(* Logix 5000 Rung export; software revision 16.03 *)

MODULES
   Local : vendor None type None code None
   mcm : vendor None type None code None
END_MODULES

TYPE MCMCONTROL :   // Stores control registers used by the processor to request special tasks from the module.
STRUCT
   WarmBoot : BOOL;   // Warm Boot
   ColdBoot : BOOL;   // Cold Boot
   SlaveControl : MCMSlaveControl;
   CmdControl : MCMCmdControl;   // Allows for a disabled command to be sent to a device (MASTER)
   EventCmd : MCMEventCmd;   // Allows a command defined in ladder to be sent to a device (MASTER)
   SlavePollStat : MCMSlavePollStatus;   // Request slave poll status for the port (MASTER).
   Passthru : MCMPassthru;   // Contains PassThru objects required when PortX.Type is set to a value between 2-4.
END_STRUCT
END_TYPE

TYPE MCMDATA :   // Contains Read Data (data read from the module to the processor) and Write Data (data written from the processor to the module)
STRUCT
   ReadData : INT[600];   // Data read from the module to the processor
   WriteData : INT[600];   // Data written from the processor to the module
END_STRUCT
END_TYPE

TYPE MCMModule :   // This object contains the information used to define the data movement between the module and the processor.
STRUCT
   WriteStartReg : INT;   // Start reg to transfer from PLC to module
   WriteRegCnt : INT;   // Number of registers to write from PLC
   ReadStartReg : INT;   // Start reg to transfer from module to PLC
   ReadRegCnt : INT;   // Number of registers to transfer from module
   BPFail : INT;   // Determines module operation if BP fails 0=continue,>0=number of retries before comm shutdown
   ErrStatPtr : INT;   // Internal DB start register for status data (-1=Ignore)
END_STRUCT
END_TYPE

TYPE MCMCONFIG :   // This object contains the data types that apply to the configuration of the module.
STRUCT
   ModDef : MCMModule;   // Module Defintion
   Port1 : MCMPort;   // Port 1 configuration settings
   Port2 : MCMPort;   // Port 2 configuration settings
   Port1MasterCmd : MCMCmd[325];   // Master commands for Port 1 (ignore if port is configured for slave mode)
   Port2MasterCmd : MCMCmd[325];   // Master commands for Port 2 (ignore if port is configured for slave mode)
END_STRUCT
END_TYPE

TYPE MCMCmdControl :   // Command Control
STRUCT
   TriggerCmdCntrl : BOOL;   // Trigger command control. User application will activate this trigger
   NumberOfCommands : INT;   // Number of commands per block (1 to 6)
   PortNumber : INT;   // MVI56-MCM Port Number of master port (1 or 2)
   CommandIndex : INT[6];   // Stores the command indexes for command control
   CmdsAddedToQueue : INT;   // Number of commands added to queue
   CmdControlBlockID : INT;   // Temporary variable to calculate control block ID
   CmdCntrlPending : BOOL;   // Auxiliary control command - prevents a second request before acknowledgment is received
END_STRUCT
END_TYPE

TYPE MCMSlaveControl :   // Special block processing for Slave Control.
STRUCT
   TriggerSlaveControl : BOOL;   // Trigger to Enable or Disable Slaves
   PortNumber : INT;   // Slave Address
   NumberOfSlaves : INT;   // Number of Slaves
   BlockNumber : INT;   // Block ID number
   SlaveIndexes : INT[200];   // Slave Indexes
   NumberOfSlavesProcessed : INT;   // Number of Slaves processed
   EnableSlaves : BOOL;   // Set 0 to Disable or 1 to Enable Slaves
END_STRUCT
END_TYPE

TYPE MCMModuleDef :   // This object contains the data types that apply to the operation of the module.
STRUCT
   CONFIG : MCMCONFIG;   // Module and port configuration
   DATA : MCMDATA;   // Modbus data transferred between module and processor
   STATUS : MCMSTATUS;   // Status information in each read block
   CONTROL : MCMCONTROL;   // Optional requests from the processor to the module
   UTIL : MCMUTIL;   // Variables for internal ladder usage - should not be accessed by user application
END_STRUCT
END_TYPE

TYPE MCMPort :   // The serial port configuration for the MVI56MCM module.
STRUCT
   Enabled : INT;   // O=Port Disabled,1=Port Enabled
   Type : INT;   // 0=Master, 1=Slave, 2=Slave: pass-through, 3=Slave: formatted pass-through/data swapped, 4=Slave: form. pass-through
   FloatFlag : INT;   // 0=No floating-point data, 1=Use floating-point data
   FloatStart : INT;   // Register offset in message for floating-point data
   FloatOffset : INT;   // Internal DB offset to start of floating-point data
   Protocol : INT;   // 0=Modbus RTU, 1=Modbus ASCII
   Baudrate : INT;   // Baudrate for port (110 to 115.2K)
   Parity : INT;   // 0=None, 1=Odd, 2=Even, 3=Mark, 4=Space
   DataBits : INT;   // 5 to 8 data bits
   StopBits : INT;   // 1 or 2 stop bits
   RTSOn : INT;   // 0-65535 mSec delay before data
   RTSOff : INT;   // 0-65535 mSec delay after data
   MinResp : INT;   // 0-65535 mSec minimum time before response to request
   UseCTS : INT;   // 0=No, 1=Yes to use CTS modem line
   SlaveID : INT;   // 1-255 Modbus Node Address (Slave)
   BitInOffset : INT;   // Internal DB offset to bit input data (Slave)
   WordInOffset : INT;   // Internal DB offset to word input data (Slave)
   OutOffset : INT;   // Internal DB offset to bit output data (Slave)
   HoldOffset : INT;   // Internal DB offset to holding register data (Slave)
   CmdCount : INT;   // Command list count (Master)
   MinCmdDelay : INT;   // 0-65535 mSec minimum time between each command (Master)
   CmdErrPtr : INT;   // Internal DB location to place command error list (Master)
   RespTO : INT;   // 0-65535 mSec response timeout for command (Master)
   RetryCount : INT;   // Retry count for failed request (Master)
   ErrorDelayCntr : INT;   // 0-65535 Command cycle count if error (Master)
   Reserved : INT;   // Reserved (Previously was UseGuardBand parameter)
   InterCharacterDelay : INT;   // 0-65535 mSec time between characters to signal end of message
   Fcn99Offset : INT;   // Internal DB offset to function 99 counter
END_STRUCT
END_TYPE

TYPE MCMSTATUS :   // This status data is returned on each read block and can be used to detect proper module operation.
STRUCT
   PassCnt : INT;   // Program cycle counter
   Product : INT[2];   // Product Name
   Rev : INT[2];   // Revision Level Number
   OP : INT[2];   // Operating Level Number
   Run : INT[2];   // Run Number
   Prt1Errs : MCMPortErrors;   // Port 1 error statistics
   Prt2Errs : MCMPortErrors;   // Port 2 error statistics
   Blk : MCMBlkStat;   // Block transfer statistics
   Port1LastErr : INT;   // Last command index that received an error on Port 1
   Port1PreviousErr : INT;   // Previous Command index that received an error on Port 1
   Port2LastErr : INT;   // Last command index that received an error on Port 2
   Port2PreviousErr : INT;   // Previous Command index that received an error on Port 2
END_STRUCT
END_TYPE

TYPE MCMBlkStat :   // This object is used to store the block transfer statistics for the module.
STRUCT
   Read : INT;   // Total number of read block transfers
   Write : INT;   // Total number of write block transfers
   Parse : INT;   // Total number of blocks parsed
   Event : INT;   // Total number of event blocks received
   Cmd : INT;   // Total number of command blocks received
   Err : INT;   // Total number of block transfer errors
END_STRUCT
END_TYPE

TYPE MCMCmd :   // This object is used to contain the attributes to define a master command. An array of these objects is used for each port.
STRUCT
   Enable : INT;   // 0=Disable,1=Continuous,2=Event Command
   IntAddress : INT;   // Module's internal address associated with the command
   PollInt : INT;   // Minimum number of seconds between issuance of command (0-65535 Sec)
   Count : INT;   // Number of registers associated with the command
   Swap : INT;   // Swap code used with command
   Node : INT;   // Node address of the target device on the network
   Func : INT;   // Function code for the command
   DevAddress : INT;   // Address in device associated with the command
END_STRUCT
END_TYPE

TYPE MCMPortErrors :   // This object is used to store the port statistics for an MVI56-MCM port.
STRUCT
   CmdReq : INT;   // Total number of command list requests sent
   CmdResp : INT;   // Total number of command list responses received
   CmdErr : INT;   // Total number of command list errors
   Requests : INT;   // Total number of requests for port
   Responses : INT;   // Total number of responses for port
   ErrSent : INT;   // Total number of errors sent
   ErrRec : INT;   // Total number of errors received
END_STRUCT
END_TYPE

TYPE MCMEventCmd :   // This object holds event command statistics.
STRUCT
   EventCmdTrigger : BOOL;   // Trigger for event command. User ladder must set this bit to initiate event command
   EventCmdPending : BOOL;   // Set after the ladder has sent an event cmd to the module and is waiting for the status to be returned
   PortNumber : INT;   // Module master port number associated to this request (1 or 2)
   SlaveAddress : INT;   // Slave target modbus address
   InternalDBAddress : INT;   // Internal database address
   PointCount : INT;   // Number of points for this command
   SwapCode : INT;   // Swap code (0= no swap, 1=swap words, 2=swap words and bytes, 3=swap bytes)
   ModbusFunctionCode : INT;   // Modbus function code
   DeviceDBAddress : INT;   // Modbus register address in target modbus slave
   EventCmdStatusReturned : INT;   // (0=Fail, 1=Sucess)
   EventBlockID : INT;   // Temporary variable to calculate event block ID
END_STRUCT
END_TYPE

TYPE MCMPassthru :   // Used to send pass-through data between the processor and the Modbus devices connected to the MVI56-MCM module.
STRUCT
   MBControl1 : CONTROL;   // Used for data to be passed through to the processor
   MBControl2 : CONTROL;   // Used for data to be passed through to the processor
   Mbdouble : DINT;   // Modbus double int tag
   MBMsg : SINT[500];   // Modbus Message
   MBMsgLen : INT;   // Modbus Offset Length
   MBOffset : INT;   // Modbus Offset
   MBOffsetBit : INT;   // Modbus Offset Bit
   MBScratch : INT[3];   // Modbus Scratch
   MBboollength : DINT;   // Holds Word size that will accommodate Coil Qty.
   MBSpecial : INT[4];   // Holds Special Function 99 data.
END_STRUCT
END_TYPE

TYPE MCMSlavePollStatus :   // This object contains all of the Slave Polling status (used when the port is used as a master)
STRUCT
   Port1Slave0Read : BOOL;   // Port 1 read slave polling status. (range 0-127)
   Port1Slave128Read : BOOL;   // Port 1 read slave polling status. (range 128-255)
   Port2Slave0Read : BOOL;   // Port 2 read slave polling status. (range 0-127)
   Port2Slave128Read : BOOL;   // Port 2 read slave polling status. (range 128-255)
   P1Slaves : INT[256];   // P1 Slave Status
   P2Slaves : INT[256];   // P2 Slave Status
END_STRUCT
END_TYPE

TYPE MCMUTIL :   // Stores tags that are used by the ladder logic for internal processing.
STRUCT
   BPLastRead : INT;   // Index of last read block
   BPLastWrite : INT;   // Index of last write block
   BlockIndex : INT;   // Computed block offset for data table
   ReadDataSize : DINT;   // Size of Read Data Array
   MaxReadBlock : DINT;   // Maximum read block
   WriteDataSize : DINT;   // Size of Write Data Array
   MaxWriteBlock : DINT;   // Maximum write block
   RBTSremainder : INT;   // Contains remainder from Read Data array size divided by the block size
   WBTSremainder : INT;   // Contains remainder from Write Data array size divided by the block size
END_STRUCT
END_TYPE

ADD_ON_INSTRUCTION AOI56MCM   (* revision 2.8, vendor ProSoft Technology Inc., ExecutePrescan *)
// This Add-On supports MVI56E-MCM modules version 3.01 and newer.
// Revision note:
// v2.8 - changes to the amount commands, now each port can support up to 325 commands.
VAR_IN_OUT
   Connection_Input : INT[250]; {required}
   Connection_Output : INT[248]; {required}
   MCM : MCMModuleDef; {required}
END_VAR
VAR
   MJFAULTS : DINT[12];
END_VAR

ROUTINE Logic   (* ladder *)
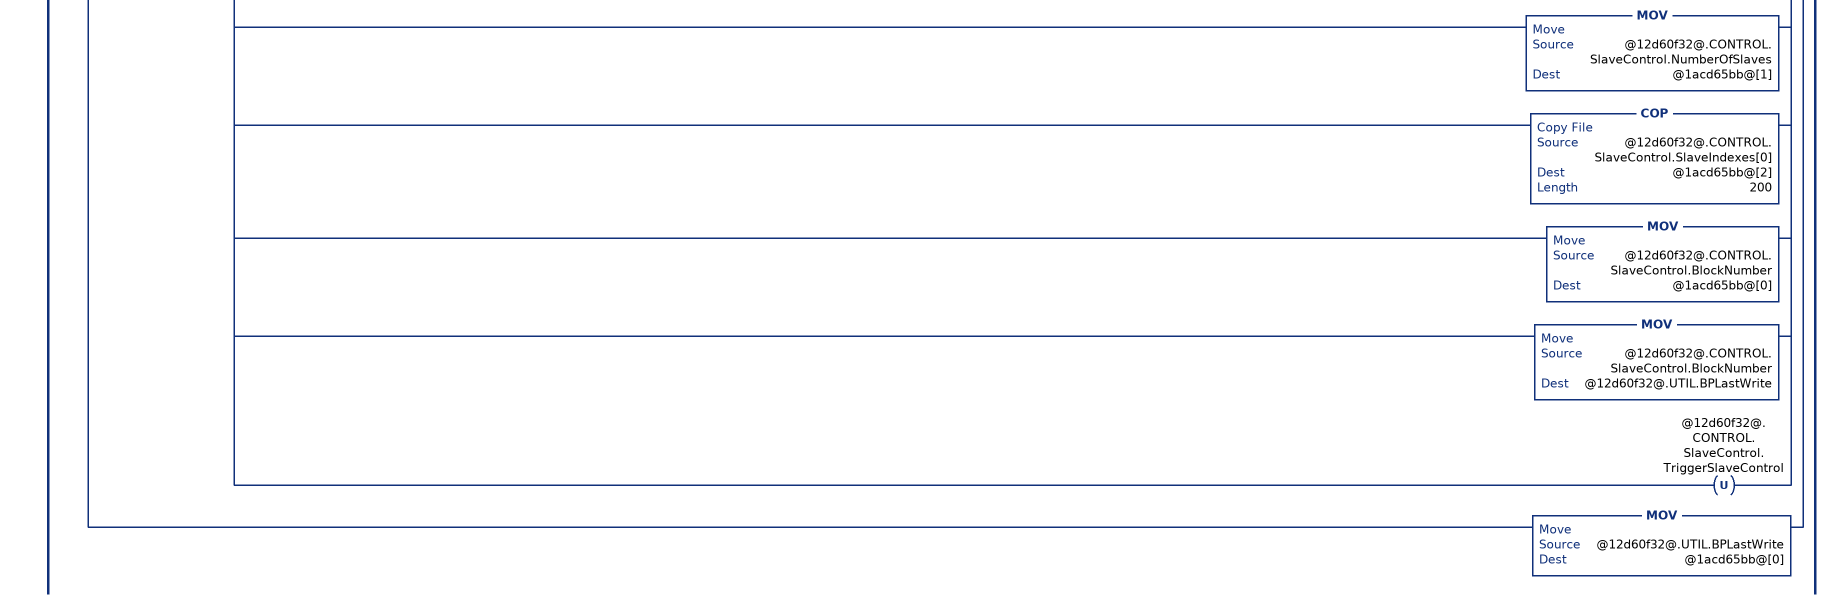
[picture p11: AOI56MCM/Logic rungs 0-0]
   0: NEQ(@c24fad98@[249],@12d60f32@.UTIL.BPLastRead)[MOV(@c24fad98@[249],@12d60f32@.UTIL.BPLastRead) ,[EQU(-1,@12d60f32@.UTIL.BPLastRead) ,EQU(0,@12d60f32@.UTIL.BPLastRead) ] [COP(@c24fad98@[202],@12d60f32@.STATUS.PassCnt,1) ,COP(@c24fad98@[203],@12d60f32@.STATUS.Product[0],8) ,COP(@c24fad98@[211],@12d60f32@.STATUS.Prt1Errs.CmdReq,7) ,COP(@c24fad98@[218],@12d60f32@.STATUS.Prt2Errs.CmdReq,7) ,COP(@c24fad98@[225],@12d60f32@.STATUS.Blk.Read,6) ,COP(@c24fad98@[231],@12d60f32@.STATUS.Port1LastErr,4) ] ,[GEQ(@12d60f32@.UTIL.BPLastRead,1) [LEQ(@12d60f32@.UTIL.BPLastRead,@12d60f32@.UTIL.MaxReadBlock) [CPT(@12d60f32@.UTIL.BlockIndex,(@12d60f32@.UTIL.BPLastRead - 1) * 200) ,COP(@c24fad98@[2],@12d60f32@.DATA.ReadData[@12d60f32@.UTIL.BlockIndex],200) ] ,CMP(@12d60f32@.UTIL.BPLastRead - @12d60f32@.UTIL.MaxReadBlock = 1) GRT(@12d60f32@.UTIL.RBTSremainder,0) [CPT(@12d60f32@.UTIL.BlockIndex,(@12d60f32@.UTIL.BPLastRead - 1) * 200) ,COP(@c24fad98@[2],@12d60f32@.DATA.ReadData[@12d60f32@.UTIL.BlockIndex],@12d60f32@.UTIL.RBTSremainder) ] ] ,COP(@c24fad98@[202],@12d60f32@.STATUS.PassCnt,1) ,COP(@c24fad98@[203],@12d60f32@.STATUS.Product[0],8) ,COP(@c24fad98@[211],@12d60f32@.STATUS.Prt1Errs.CmdReq,7) ,COP(@c24fad98@[218],@12d60f32@.STATUS.Prt2Errs.CmdReq,7) ,COP(@c24fad98@[225],@12d60f32@.STATUS.Blk.Read,6) ,COP(@c24fad98@[231],@12d60f32@.STATUS.Port1LastErr,4) ] ,EQU(9996,@12d60f32@.UTIL.BPLastRead) [MOV(@c24fad98@[2],@12d60f32@.CONTROL.Passthru.MBMsgLen) ,COP(@c24fad98@[4],@12d60f32@.CONTROL.Passthru.MBMsg[0],@12d60f32@.CONTROL.Passthru.MBMsgLen) ] ,LIM(9956,@12d60f32@.UTIL.BPLastRead,9957) [MOV(@c24fad98@[3],@12d60f32@.CONTROL.Passthru.MBOffset) ,LES(@12d60f32@.CONTROL.Passthru.MBOffset,@12d60f32@.UTIL.WriteDataSize) COP(@c24fad98@[4],@12d60f32@.DATA.WriteData[@12d60f32@.CONTROL.Passthru.MBOffset],@c24fad98@[2]) ] ,EQU(9958,@12d60f32@.UTIL.BPLastRead) [MOV(@c24fad98@[3],@12d60f32@.CONTROL.PassThru.MBOffsetBit) ,MOV(@c24fad98@[4],@12d60f32@.CONTROL.PassThru.MBScratch[2]) ,DIV(@12d60f32@.CONTROL.PassThru.MBOffsetBit,16,@12d60f32@.CONTROL.PassThru.MBOffset) ,MOD(@12d60f32@.CONTROL.PassThru.MBOffsetBit,16,@12d60f32@.CONTROL.PassThru.MBOffsetBit) ,XPY(2,@12d60f32@.CONTROL.PassThru.MBOffsetBit,@12d60f32@.CONTROL.PassThru.mbdouble) ,MVM(@12d60f32@.CONTROL.PassThru.mbdouble,16#0000_ffff,@12d60f32@.CONTROL.PassThru.MBOffsetBit) ,GEQ(@12d60f32@.CONTROL.PassThru.MBOffset,0) LES(@12d60f32@.CONTROL.PassThru.MBOffset,@12d60f32@.UTIL.WriteDataSize) LEQ(@12d60f32@.CONTROL.PassThru.MBOffset,2048) [NEQ(@12d60f32@.CONTROL.PassThru.MBScratch[2],0) OR(@12d60f32@.CONTROL.PassThru.MBOffsetBit,@12d60f32@.DATA.WriteData[@12d60f32@.CONTROL.PassThru.MBOffset],@12d60f32@.DATA.WriteData[@12d60f32@.CONTROL.PassThru.MBOffset]) ,EQU(@12d60f32@.CONTROL.PassThru.MBScratch[2],0) [NOT(@12d60f32@.CONTROL.PassThru.MBOffsetBit,@12d60f32@.CONTROL.PassThru.MBOffsetBit) ,AND(@12d60f32@.CONTROL.PassThru.MBOffsetBit,@12d60f32@.DATA.WriteData[@12d60f32@.CONTROL.PassThru.MBOffset],@12d60f32@.DATA.WriteData[@12d60f32@.CONTROL.PassThru.MBOffset]) ] ] ] ,EQU(9959,@12d60f32@.UTIL.BPLastRead) [MOV(@c24fad98@[3],@12d60f32@.CONTROL.Passthru.MBOffset) ,MOV(@c24fad98@[2],@12d60f32@.CONTROL.Passthru.MBControl1.LEN) ,MOV(@c24fad98@[2],@12d60f32@.CONTROL.Passthru.MBControl2.LEN) ,FAL(@12d60f32@.CONTROL.Passthru.MBControl1,?,?,ALL,@12d60f32@.DATA.WriteData[@12d60f32@.CONTROL.Passthru.MBOffset+@12d60f32@.CONTROL.Passthru.MBControl1.POS],@12d60f32@.DATA.WriteData[@12d60f32@.CONTROL.Passthru.MBOffset+@12d60f32@.CONTROL.Passthru.MBControl1.POS] AND(NOT @c24fad98@[54+@12d60f32@.CONTROL.Passthru.MBControl1.POS])) ,FAL(@12d60f32@.CONTROL.Passthru.MBControl2,?,?,ALL,@12d60f32@.DATA.WriteData[@12d60f32@.CONTROL.Passthru.MBOffset+@12d60f32@.CONTROL.Passthru.MBControl2.POS],@12d60f32@.DATA.WriteData[@12d60f32@.CONTROL.Passthru.MBOffset+@12d60f32@.CONTROL.Passthru.MBControl2.POS] OR(@c24fad98@[54+@12d60f32@.CONTROL.Passthru.MBControl2.POS] AND @c24fad98@[4+@12d60f32@.CONTROL.Passthru.MBControl2.POS])) ,RES(@12d60f32@.CONTROL.Passthru.MBControl1) ,RES(@12d60f32@.CONTROL.Passthru.MBControl2) ] ,LIM(3002,@12d60f32@.UTIL.BPLastRead,3003) [CPT(@12d60f32@.UTIL.BlockIndex,(@12d60f32@.UTIL.BPLastRead-3002)*128) ,COP(@c24fad98@[2],@12d60f32@.CONTROL.SlavePollStat.P1Slaves[@12d60f32@.UTIL.BlockIndex],128) ] ,LIM(3102,@12d60f32@.UTIL.BPLastRead,3103) [CPT(@12d60f32@.UTIL.BlockIndex,(@12d60f32@.UTIL.BPLastRead-3102)*128) ,COP(@c24fad98@[2],@12d60f32@.CONTROL.SlavePollStat.P2Slaves[@12d60f32@.UTIL.BlockIndex],128) ] ,[LIM(5001,@12d60f32@.UTIL.BPLastRead,5006) ,LIM(5101,@12d60f32@.UTIL.BPLastRead,5106) ] [MOV(@c24fad98@[2],@12d60f32@.CONTROL.CmdControl.CmdsAddedToQueue) ,OTU(@12d60f32@.CONTROL.CmdControl.CmdCntrlPending) ,OTU(@12d60f32@.CONTROL.CmdControl.TriggerCmdCntrl) ] ,[LIM(1000,@12d60f32@.UTIL.BPLastRead,1255) ,LIM(2000,@12d60f32@.UTIL.BPLastRead,2255) ] [MOV(@c24fad98@[2],@12d60f32@.CONTROL.EventCmd.EventCmdStatusReturned) ,OTU(@12d60f32@.CONTROL.EventCmd.EventCmdPending) ,OTU(@12d60f32@.CONTROL.EventCmd.EventCmdTrigger) ] ,EQU(-9000,@12d60f32@.UTIL.BPLastRead) [COP(@c24fad98@[2],@12d60f32@.CONFIG.ModDef.WriteStartReg,6) ,COP(@c24fad98@[8],@12d60f32@.CONFIG.Port1.Enabled,25) ,COP(@c24fad98@[33],@12d60f32@.CONFIG.Port2.Enabled,25) ,COP(@c24fad98@[58],@12d60f32@.CONFIG.Port1.Reserved,3) ,COP(@c24fad98@[61],@12d60f32@.CONFIG.Port2.Reserved,3) ,MOV(@12d60f32@.UTIL.BPLastRead,@1acd65bb@[0]) ] ,LIM(-6012,@12d60f32@.UTIL.BPLastRead,-6000) [CPT(@12d60f32@.UTIL.BPLastWrite,(-@12d60f32@.UTIL.BPLastRead-6000)*25) ,COP(@c24fad98@[2],@12d60f32@.CONFIG.Port1MasterCmd[@12d60f32@.UTIL.BPLastWrite].Enable,200) ,MOV(@12d60f32@.UTIL.BPLastRead,@1acd65bb@[0]) ] ,LIM(-6112,@12d60f32@.UTIL.BPLastRead,-6100) [CPT(@12d60f32@.UTIL.BPLastWrite,(-@12d60f32@.UTIL.BPLastRead-6100)*25) ,COP(@c24fad98@[2],@12d60f32@.CONFIG.Port2MasterCmd[@12d60f32@.UTIL.BPLastWrite].Enable,200) ,MOV(@12d60f32@.UTIL.BPLastRead,@1acd65bb@[0]) ] ,MOV(@c24fad98@[1],@12d60f32@.UTIL.BPLastWrite) ,XIC(@12d60f32@.CONTROL.WarmBoot) [MOV(9998,@12d60f32@.UTIL.BPLastWrite) ,OTU(@12d60f32@.CONTROL.WarmBoot) ] ,XIC(@12d60f32@.CONTROL.ColdBoot) [MOV(9999,@12d60f32@.UTIL.BPLastWrite) ,OTU(@12d60f32@.CONTROL.ColdBoot) ] ,GEQ(@12d60f32@.UTIL.BPLastWrite,1) [LEQ(@12d60f32@.UTIL.BPLastWrite,@12d60f32@.UTIL.MaxWriteBlock) [CPT(@12d60f32@.UTIL.BlockIndex,(@12d60f32@.UTIL.BPLastWrite - 1) * 200) ,COP(@12d60f32@.DATA.WriteData[@12d60f32@.UTIL.BlockIndex],@1acd65bb@[1],200) ] ,CMP(@12d60f32@.UTIL.BPLastWrite - @12d60f32@.UTIL.MaxWriteBlock = 1) GRT(@12d60f32@.UTIL.WBTSremainder,0) [CPT(@12d60f32@.UTIL.BlockIndex,(@12d60f32@.UTIL.BPLastWrite - 1) * 200) ,COP(@12d60f32@.DATA.WriteData[@12d60f32@.UTIL.BlockIndex],@1acd65bb@[1],@12d60f32@.UTIL.WBTSremainder) ] ] ,EQU(9000,@12d60f32@.UTIL.BPLastWrite) [COP(@12d60f32@.CONFIG.ModDef.WriteStartReg,@1acd65bb@[1],6) ,COP(@12d60f32@.CONFIG.Port1.Enabled,@1acd65bb@[7],25) ,COP(@12d60f32@.CONFIG.Port2.Enabled,@1acd65bb@[32],25) ,COP(@12d60f32@.CONFIG.Port1.Reserved,@1acd65bb@[57],3) ,COP(@12d60f32@.CONFIG.Port2.Reserved,@1acd65bb@[60],3) ] ,LIM(6000,@12d60f32@.UTIL.BPLastWrite,6012) [CPT(@12d60f32@.UTIL.BlockIndex,(@12d60f32@.UTIL.BPLastWrite-6000)*25) ,COP(@12d60f32@.CONFIG.Port1MasterCmd[@12d60f32@.UTIL.BlockIndex].Enable,@1acd65bb@[1],200) ] ,LIM(6100,@12d60f32@.UTIL.BPLastWrite,6112) [CPT(@12d60f32@.UTIL.BlockIndex,(@12d60f32@.UTIL.BPLastWrite-6100)*25) ,COP(@12d60f32@.CONFIG.Port2MasterCmd[@12d60f32@.UTIL.BlockIndex].Enable,@1acd65bb@[1],200) ] ,XIC(@12d60f32@.CONTROL.SlavePollStat.Port1Slave0Read) [MOV(3002,@12d60f32@.UTIL.BPLastWrite) ,OTU(@12d60f32@.CONTROL.SlavePollStat.Port1Slave0Read) ] ,XIC(@12d60f32@.CONTROL.SlavePollStat.Port1Slave128Read) [MOV(3003,@12d60f32@.UTIL.BPLastWrite) ,OTU(@12d60f32@.CONTROL.SlavePollStat.Port1Slave128Read) ] ,XIC(@12d60f32@.CONTROL.SlavePollStat.Port2Slave0Read) [MOV(3102,@12d60f32@.UTIL.BPLastWrite) ,OTU(@12d60f32@.CONTROL.SlavePollStat.Port2Slave0Read) ] ,XIC(@12d60f32@.CONTROL.SlavePollStat.Port2Slave128Read) [MOV(3103,@12d60f32@.UTIL.BPLastWrite) ,OTU(@12d60f32@.CONTROL.SlavePollStat.Port2Slave128Read) ] ,XIC(@12d60f32@.CONTROL.CmdControl.TriggerCmdCntrl) XIO(@12d60f32@.CONTROL.CmdControl.CmdCntrlPending) [COP(@12d60f32@.CONTROL.CmdControl.CommandIndex[0],@1acd65bb@[1],6) ,ADD(5000,@12d60f32@.CONTROL.CmdControl.NumberOfCommands,@12d60f32@.CONTROL.CmdControl.CmdControlBlockID) ,EQU(@12d60f32@.CONTROL.CmdControl.PortNumber,2) ADD(100,@12d60f32@.CONTROL.CmdControl.CmdControlBlockID,@12d60f32@.CONTROL.CmdControl.CmdControlBlockID) ,MOV(@12d60f32@.CONTROL.CmdControl.CmdControlBlockID,@12d60f32@.UTIL.BPLastWrite) ,OTL(@12d60f32@.CONTROL.CmdControl.CmdCntrlPending) ] ,XIC(@12d60f32@.CONTROL.EventCmd.EventCmdTrigger) XIO(@12d60f32@.CONTROL.EventCmd.EventCmdPending) [COP(@12d60f32@.CONTROL.EventCmd.InternalDBAddress,@1acd65bb@[1],5) ,ADD(1000,@12d60f32@.CONTROL.EventCmd.SlaveAddress,@12d60f32@.CONTROL.EventCmd.EventBlockID) ,EQU(@12d60f32@.CONTROL.EventCmd.PortNumber,2) ADD(@12d60f32@.CONTROL.EventCmd.EventBlockID,1000,@12d60f32@.CONTROL.EventCmd.EventBlockID) ,MOV(@12d60f32@.CONTROL.EventCmd.EventBlockID,@12d60f32@.UTIL.BPLastWrite) ,OTL(@12d60f32@.CONTROL.EventCmd.EventCmdPending) ] ,[LIM(3000,@c24fad98@[249],3001) ,LIM(3100,@c24fad98@[249],3101) ] MOV(@c24fad98@[2],@12d60f32@.CONTROL.SlaveControl.NumberOfSlavesProcessed) ,XIC(@12d60f32@.CONTROL.SlaveControl.TriggerSlaveControl) [MOV(3000,@12d60f32@.CONTROL.SlaveControl.BlockNumber) ,EQU(@12d60f32@.CONTROL.SlaveControl.PortNumber,2) ADD(100,@12d60f32@.CONTROL.SlaveControl.BlockNumber,@12d60f32@.CONTROL.SlaveControl.BlockNumber) ,XIC(@12d60f32@.CONTROL.SlaveControl.EnableSlaves) ADD(1,@12d60f32@.CONTROL.SlaveControl.BlockNumber,@12d60f32@.CONTROL.SlaveControl.BlockNumber) ,MOV(@12d60f32@.CONTROL.SlaveControl.NumberOfSlaves,@1acd65bb@[1]) ,COP(@12d60f32@.CONTROL.SlaveControl.SlaveIndexes[0],@1acd65bb@[2],200) ,MOV(@12d60f32@.CONTROL.SlaveControl.BlockNumber,@1acd65bb@[0]) ,MOV(@12d60f32@.CONTROL.SlaveControl.BlockNumber,@12d60f32@.UTIL.BPLastWrite) ,OTU(@12d60f32@.CONTROL.SlaveControl.TriggerSlaveControl) ] ,MOV(@12d60f32@.UTIL.BPLastWrite,@1acd65bb@[0]) ];
END_ROUTINE

ROUTINE Prescan   (* ladder *)
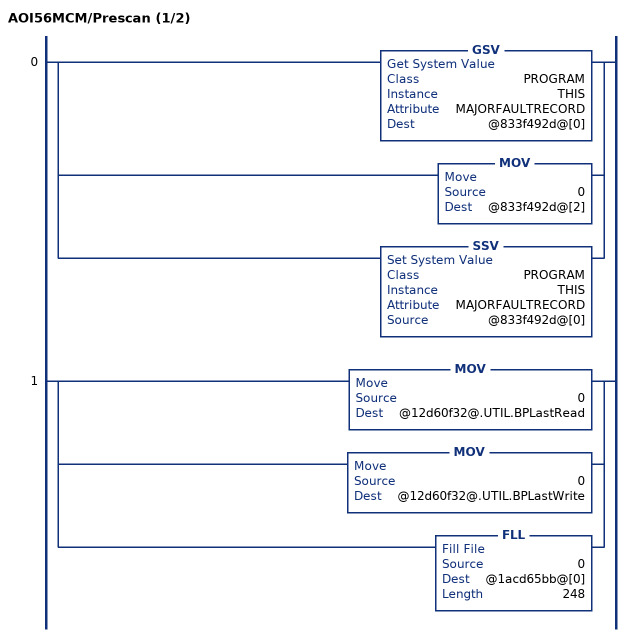
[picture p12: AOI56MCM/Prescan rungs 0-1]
   0: [GSV(PROGRAM,THIS,MAJORFAULTRECORD,@833f492d@[0]) ,MOV(0,@833f492d@[2]) ,SSV(PROGRAM,THIS,MAJORFAULTRECORD,@833f492d@[0]) ];
   1: [MOV(0,@12d60f32@.UTIL.BPLastRead) ,MOV(0,@12d60f32@.UTIL.BPLastWrite) ,FLL(0,@1acd65bb@[0],248) ];
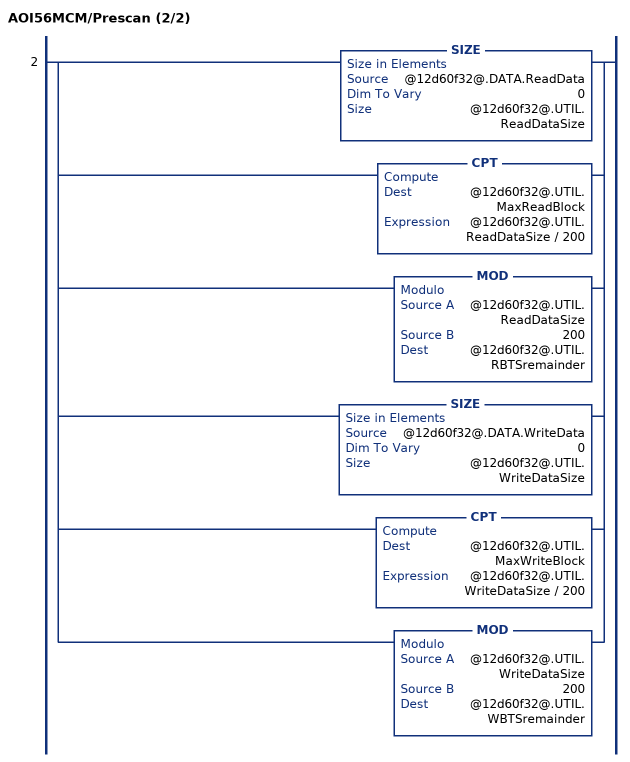
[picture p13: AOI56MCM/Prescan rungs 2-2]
   2: [SIZE(@12d60f32@.DATA.ReadData,0,@12d60f32@.UTIL.ReadDataSize) ,CPT(@12d60f32@.UTIL.MaxReadBlock,@12d60f32@.UTIL.ReadDataSize / 200) ,MOD(@12d60f32@.UTIL.ReadDataSize,200,@12d60f32@.UTIL.RBTSremainder) ,SIZE(@12d60f32@.DATA.WriteData,0,@12d60f32@.UTIL.WriteDataSize) ,CPT(@12d60f32@.UTIL.MaxWriteBlock,@12d60f32@.UTIL.WriteDataSize / 200) ,MOD(@12d60f32@.UTIL.WriteDataSize,200,@12d60f32@.UTIL.WBTSremainder) ];
END_ROUTINE
END_ADD_ON_INSTRUCTION

VAR_GLOBAL   (* controller tags *)
   MCM : MCMModuleDef;
   AOI56MCM : AOI56MCM;
   Local:1:I : AB:1756_MODULE_INT_500Bytes:I:0;
   Local:1:O : AB:1756_MODULE_INT_496Bytes:O:0;
END_VAR

PROGRAM MainProgram

ROUTINE MainRoutine   (* ladder *)
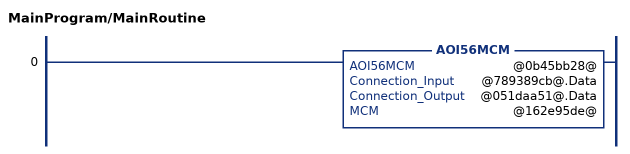
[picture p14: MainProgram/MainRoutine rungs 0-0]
   0: AOI56MCM(@0b45bb28@,@789389cb@.Data,@051daa51@.Data,@162e95de@);
END_ROUTINE
END_PROGRAM
